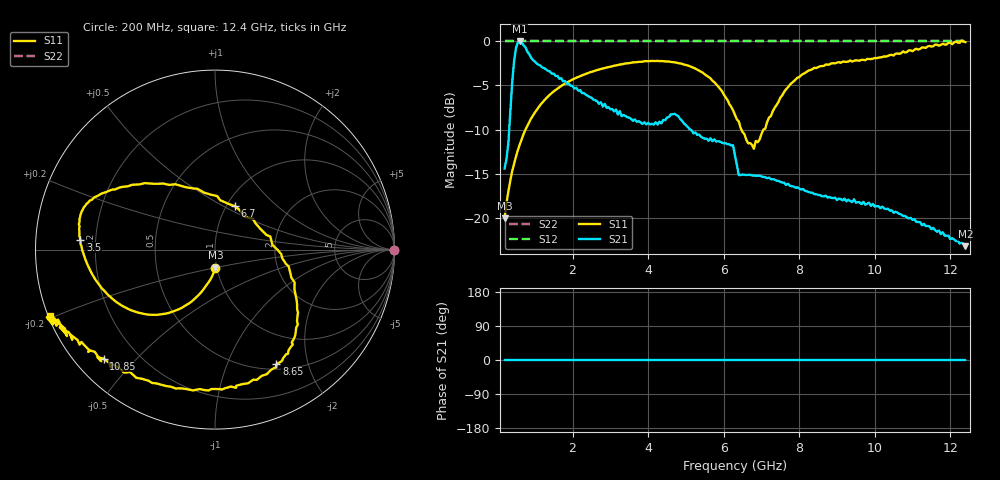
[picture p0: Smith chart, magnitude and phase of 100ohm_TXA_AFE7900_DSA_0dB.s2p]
# hz S db R 100
! AFE7900 - TX Channel A, DSA = 0dB, Fs = 11.79648 GHz
! 4/8/20
! Port 1 - SE representation of DAC differential output
! Port 2 - DAC analogoutput
! freq  dbS11  angS11
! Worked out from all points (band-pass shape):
!   245 points, 200 MHz to 12.4 GHz, reference 100 ohm
!   highest |S21| = 0.02 dB at 600 MHz (marker M1); lowest = -23.2 dB at 12.4 GHz (marker M2)
!   |S21| within 3 dB of the highest: 435.3 MHz to 1.21 GHz (774.6 MHz wide, 94.2 % of centre)
!   lowest |S11| = -20.0 dB at 200 MHz (marker M3), VSWR 1.22, Z = 98.5 - j19.9 ohm
!   |S11| at or under -10 dB: start of sweep to 751.6 MHz; 6.471 GHz to 7.049 GHz (578 MHz wide, 8.55 % of centre)
!   |S22| runs from 0.0 to 0.0 dB; largest |S21 - S12| = 0.93
!   S11 on the Smith chart (normalised r, x): 200 MHz: 0.98, -0.20; 3.5 GHz: 0.14, +0.04; 6.7 GHz: 1.09, +0.57; 8.65 GHz: 0.57, -1.52; 10.85 GHz: 0.08, -0.41; 12.4 GHz: 0.01, -0.19
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2e8  -19.99 -88.7  -14.38 0.0  0.00 0.0  0.00 0.0
3e8  -16.96 -95.3  -11.47 0.0  0.00 0.0  0.00 0.0
4.5e8  -13.87 -103.4  -2.27 0.0  0.00 0.0  0.00 0.0
5e8  -13.05 -105.4  -0.78 0.0  0.00 0.0  0.00 0.0
6e8  -11.68 -109.0  0.02 0.0  0.00 0.0  0.00 0.0
1.05e9  -7.75 -123.5  -2.52 0.0  0.00 0.0  0.00 0.0
2.25e9  -3.85 -156.1  -5.85 0.0  0.00 0.0  0.00 0.0
3.5e9  -2.47 175.8  -8.63 0.0  0.00 0.0  0.00 0.0
4.3e9  -2.24 164.8  -9.09 0.0  0.00 0.0  0.00 0.0
4.7e9  -2.38 160.4  -8.20 0.0  0.00 0.0  0.00 0.0
5.45e9  -3.56 149.8  -10.92 0.0  0.00 0.0  0.00 0.0
6.3e9  -8.32 115.1  -12.94 0.0  0.00 0.0  0.00 0.0
6.4e9  -9.06 106.0  -15.12 0.0  0.00 0.0  0.00 0.0
6.7e9  -11.51 65.5  -15.09 0.0  0.00 0.0  0.00 0.0
7.5e9  -6.38 -22.4  -15.89 0.0  0.00 0.0  0.00 0.0
8.35e9  -3.15 -54.0  -17.12 0.0  0.00 0.0  0.00 0.0
8.65e9  -2.80 -61.8  -17.54 0.0  0.00 0.0  0.00 0.0
9.5e9  -2.15 -87.3  -18.23 0.0  0.00 0.0  0.00 0.0
1.04e10  -1.57 -120.9  -19.14 0.0  0.00 0.0  0.00 0.0
1.085e10  -1.23 -135.6  -19.90 0.0  0.00 0.0  0.00 0.0
1.16e10  -0.37 -151.9  -21.36 0.0  0.00 0.0  0.00 0.0
1.24e10  -0.10 -158.2  -23.16 0.0  0.00 0.0  0.00 0.0
